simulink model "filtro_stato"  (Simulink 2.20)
settings: Solver=VariableStepDiscrete  StartTime=0.0  StopTime=50.0  RelTol=1e-3  AbsTol=1e-6
undefined symbols (not defined in the file or in its folder): k1, k2, T
libraries: simulink x2

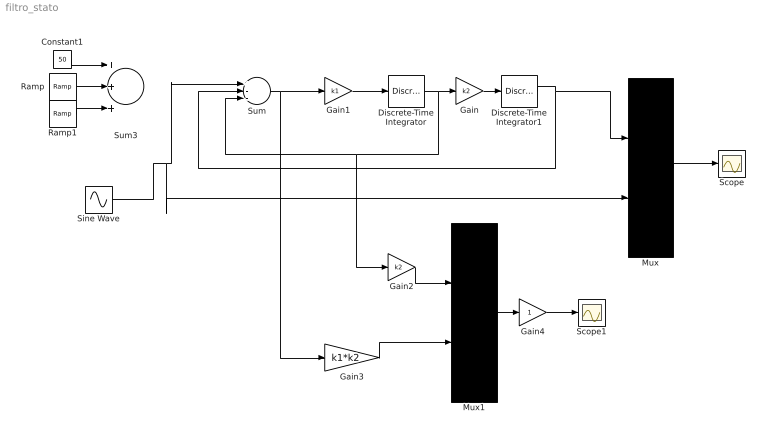
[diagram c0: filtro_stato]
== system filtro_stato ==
  Constant1 : Constant  Value=50
  Discrete-Time Integrator : DiscreteIntegrator  IntegratorMethod=ForwardEuler  ExternalReset=none  InitialConditionSource=internal  InitialCondition=0  LimitOutput=off  UpperSaturationLimit=inf  LowerSaturationLimit=-inf  ShowSaturationPort=off  ShowStatePort=off  SampleTime=T
  Discrete-Time Integrator1 : DiscreteIntegrator  IntegratorMethod=ForwardEuler  ExternalReset=none  InitialConditionSource=internal  InitialCondition=0  LimitOutput=off  UpperSaturationLimit=inf  LowerSaturationLimit=-inf  ShowSaturationPort=off  ShowStatePort=off  SampleTime=T
  Gain : Gain  Gain=k2
  Gain1 : Gain  Gain=k1
  Gain2 : Gain  Gain=k2
  Gain3 : Gain  Gain=k1*k2
  Gain4 : Gain  Gain=1
  Mux : Mux  Inputs=2
  Mux1 : Mux  Inputs=2
  Ramp : simulink/Sources/Ramp  slope=-50  start=10  X0=0
  Ramp1 : simulink/Sources/Ramp  slope=+100  start=20  X0=0
  Scope : Scope
  Scope1 : Scope
  Sine Wave : Sin  Amplitude=50  Frequency=0.5  Phase=0  SampleTime=0
  Sum : Sum  Inputs=+--
  Sum3 : Sum  Inputs=+++
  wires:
  Constant1/1 -> Sum3/1
  Ramp/1 -> Sum3/2
  Ramp1/1 -> Sum3/3
  Discrete-Time Integrator/1 -> Sum/3, Gain2/1, Gain/1
  Mux/1 -> Scope/1
  Gain2/1 -> Mux1/1
  Gain1/1 -> Discrete-Time Integrator/1
  Sum/1 -> Gain1/1, Gain3/1
  Gain3/1 -> Mux1/2
  Sine Wave/1 -> Sum/1, Mux/2
  Mux1/1 -> Gain4/1
  Gain4/1 -> Scope1/1
  Discrete-Time Integrator1/1 -> Sum/2, Mux/1
  Gain/1 -> Discrete-Time Integrator1/1
